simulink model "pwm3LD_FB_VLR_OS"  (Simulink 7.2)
settings: Solver=ode3  SolverMode=SingleTasking  StartTime=0.0  StopTime=0.1  FixedStep=10e-6  MaxStep=1e-4  RelTol=1e-3
PreLoadFcn:
  | INIT_PWM_3L

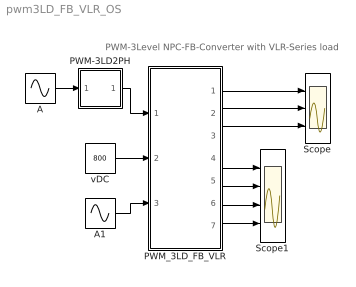
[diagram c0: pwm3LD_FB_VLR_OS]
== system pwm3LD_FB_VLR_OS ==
  note: PWM-3Level NPC-FB-Converter with VLR-Series load
  A : Sin  Amplitude=.8  Frequency=2*pi*50  Phase=[0 ]  SampleTime=0
  A1 : Sin  Amplitude=200  Frequency=2*pi*50  Phase=[0 ]  SampleTime=0
  PWM-3LD2PH : Subsystem  mask(PWM-3LD_3PH){FT=900, PHT=0, A=0.5, O1=0.5, O2=-0.5, DT=1e-6}
      mask prompts: FT "Frequency of Trian Sig."; PHT "Phase Angle of Trian. Sig."; A "Amplitude of Trian. Sig."; O1 "Offset of 1st Trian"; O2 "Offset of 2nd Trian."; DT "Dead Time"
      mask help: Pulse Width Modulation for 2 Legs of 3 Level Neutral point clamped Converter
  PWM_3LD_FB_VLR : Subsystem  mask(pwm_3LD_FB_VLR_OS){RL=1, LL=1e-3}
      mask prompts: RL "Load Resistance"; LL "Load Inductance"
      mask help: Open Source 3-Level NPC Full Bridge Converter with VLR load Input Vector u: u[0]= L3L1_TD1.gate u[1]= L3L1_TD2.gate u[2]= L3L1_TD3.gate u[3]= L3L1_TD4.gate u[4]= L3L2_TD1.gate u[5]= L3L2_TD2.gate u[6]= L3L2_TD3.gate u[7]= L3L2_TD4.gate u[8]= VDC u[9]= EL Output Vector y: y[0]= Va.v, Output AC Voltage to middle point y[1]= Ia.I, Output AC Current y[2]= Vab.V, Output AC Voltage y[3]= T1.I y[4]= D1.I y[5]= T1.V y[6]= T2.I y[7]= D2.I y[8]= T2.V y[9]= D5.I y[10]= D5.V y[11]= IDC1, Input DC Current y[12]= IDC2, Input DC Current Parameter Vector p: p[0]=RL p[1]=LL You can pause the simulation during 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
  Scope : Scope  NumInputPorts=3
  Scope1 : Scope  NumInputPorts=4
  vDC : Constant  Value=800  OutDataType=sfix(16)  OutScaling=2^0
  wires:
  A/1 -> PWM-3LD2PH/1(In1)
  vDC/1 -> PWM_3LD_FB_VLR/2(vDC)
  A1/1 -> PWM_3LD_FB_VLR/3(E_A)
  PWM-3LD2PH/1(Out1) -> PWM_3LD_FB_VLR/1(Sw)
  PWM_3LD_FB_VLR/4("iT1, iD1,vT1") -> Scope1/1
  PWM_3LD_FB_VLR/5("iT2, iD2,vT2") -> Scope1/2
  PWM_3LD_FB_VLR/6(iD5,vD5) -> Scope1/3
  PWM_3LD_FB_VLR/7(iDC1,iDC2) -> Scope1/4
  PWM_3LD_FB_VLR/1(vA) -> Scope/1
  PWM_3LD_FB_VLR/2(iA) -> Scope/2
  PWM_3LD_FB_VLR/3(vAB) -> Scope/3

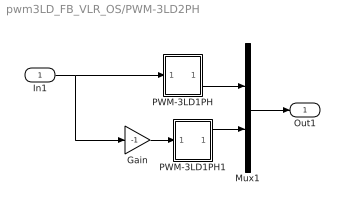
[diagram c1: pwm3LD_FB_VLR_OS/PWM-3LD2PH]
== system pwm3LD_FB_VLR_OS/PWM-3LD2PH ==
  In1 : Inport  OutDataType=sfix(16)  OutScaling=2^0
  Gain : Gain  Gain=-1  ParameterDataType=sfix(16)  ParameterScaling=2^0  OutDataType=sfix(16)  OutScaling=2^0
  Mux1 : Mux  Inputs=2
  PWM-3LD1PH : Subsystem  mask(PWM-3LD1PH){FT=FT, PHT=PHT, A=A, O1=O1, O2=O2, DT=DT}
      mask prompts: FT "Frequency of Trian Sig."; PHT "Phase Angle of Trian. Sig."; A "Amplitude of Trian. Sig."; O1 "Offset of 1st Trian"; O2 "Offset of 2nd Trian."; DT "Dead Time"
      mask help: Pulse Width Modulation for 1 Phase 3 Level Floating Capacitor Converter
  PWM-3LD1PH1 : Subsystem  mask(PWM-3LD1PH){FT=FT, PHT=PHT, A=A, O1=O1, O2=O2, DT=DT}
      mask prompts: FT "Frequency of Trian Sig."; PHT "Phase Angle of Trian. Sig."; A "Amplitude of Trian. Sig."; O1 "Offset of 1st Trian"; O2 "Offset of 2nd Trian."; DT "Dead Time"
      mask help: Pulse Width Modulation for 1 Phase 3 Level Floating Capacitor Converter
  Out1 : Outport
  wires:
  PWM-3LD1PH1/1(Out1) -> Mux1/2
  PWM-3LD1PH/1(Out1) -> Mux1/1
  In1/1 -> Gain/1, PWM-3LD1PH/1(In1)
  Gain/1 -> PWM-3LD1PH1/1(In1)
  Mux1/1 -> Out1/1

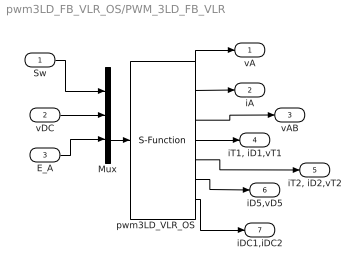
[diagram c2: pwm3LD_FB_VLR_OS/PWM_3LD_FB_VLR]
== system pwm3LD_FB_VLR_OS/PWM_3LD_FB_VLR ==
  Sw : Inport  OutDataType=sfix(16)  OutScaling=2^0
  vDC : Inport  Port=2  OutDataType=sfix(16)  OutScaling=2^0
  E_A : Inport  Port=3  OutDataType=sfix(16)  OutScaling=2^0
  Mux : Mux  Inputs="[8  1  1]"
  pwm3LD_VLR_OS : S-Function  FunctionName=s_pwm_3LD_FB_VLR_OS  Parameters="[RL  LL]"  EnableBusSupport=off
  vA : Outport  OutDataType=sfix(16)  OutScaling=2^0
  iA : Outport  Port=2  OutDataType=sfix(16)  OutScaling=2^0
  vAB : Outport  Port=3  OutDataType=sfix(16)  OutScaling=2^0
  "iT1, iD1,vT1" : Outport  Port=4  OutDataType=sfix(16)  OutScaling=2^0
  "iT2, iD2,vT2" : Outport  Port=5  OutDataType=sfix(16)  OutScaling=2^0
  iD5,vD5 : Outport  Port=6  OutDataType=sfix(16)  OutScaling=2^0
  iDC1,iDC2 : Outport  Port=7  OutDataType=sfix(16)  OutScaling=2^0
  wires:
  Sw/1 -> Mux/1
  vDC/1 -> Mux/2
  Mux/1 -> pwm3LD_VLR_OS/1
  E_A/1 -> Mux/3
  pwm3LD_VLR_OS/1 -> vA/1
  pwm3LD_VLR_OS/2 -> iA/1
  pwm3LD_VLR_OS/3 -> vAB/1
  pwm3LD_VLR_OS/4 -> "iT1, iD1,vT1"/1
  pwm3LD_VLR_OS/5 -> "iT2, iD2,vT2"/1
  pwm3LD_VLR_OS/6 -> iD5,vD5/1
  pwm3LD_VLR_OS/7 -> iDC1,iDC2/1

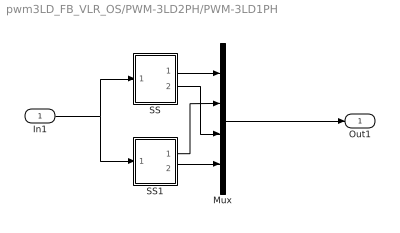
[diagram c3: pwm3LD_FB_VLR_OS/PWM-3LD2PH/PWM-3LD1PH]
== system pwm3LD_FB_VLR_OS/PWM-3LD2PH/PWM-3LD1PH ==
  In1 : Inport  OutDataType=sfix(16)  OutScaling=2^0
  Mux : Mux
  SS : Subsystem
  SS1 : Subsystem
  Out1 : Outport
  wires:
  In1/1 -> SS1/1(I1), SS/1(I1)
  SS1/1(O1) -> Mux/2
  SS/2(O2) -> Mux/3
  Mux/1 -> Out1/1
  SS/1(O1) -> Mux/1
  SS1/2(O2) -> Mux/4

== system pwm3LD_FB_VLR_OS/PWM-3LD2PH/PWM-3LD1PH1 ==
  In1 : Inport  OutDataType=sfix(16)  OutScaling=2^0
  Mux : Mux
  SS : Subsystem
  SS1 : Subsystem
  Out1 : Outport
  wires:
  SS1/2(O2) -> Mux/4
  SS/1(O1) -> Mux/1
  Mux/1 -> Out1/1
  SS/2(O2) -> Mux/3
  SS1/1(O1) -> Mux/2
  In1/1 -> SS/1(I1), SS1/1(I1)

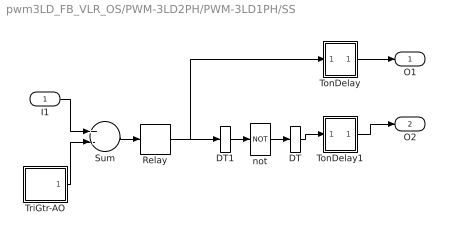
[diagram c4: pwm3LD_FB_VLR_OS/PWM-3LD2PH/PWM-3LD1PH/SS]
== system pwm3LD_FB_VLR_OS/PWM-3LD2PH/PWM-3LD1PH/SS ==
  I1 : Inport  OutDataType=sfix(16)  OutScaling=2^0
  DT : DataTypeConversion
  DT1 : DataTypeConversion
  Relay : Relay  OutDataType=sfix(16)  OutScaling=2^0
  Sum : Sum  Inputs=+-  OutDataType=sfix(16)  OutScaling=2^0
  TonDelay : Subsystem  mask(TonDelay){DT=DT}
      mask prompts: DT "Dead Time"
      mask help: Turn on dead time to protect against short circuit of the converter leg
  TonDelay1 : Subsystem  mask(TonDelay){DT=DT}
      mask prompts: DT "Dead Time"
      mask help: Turn on dead time to protect against short circuit of the converter leg
  TriGtr-AO : Subsystem  mask(TriGtr-AO){A=A, O=O1, T=1/FT, Td=PHT/FT/180}
      mask prompts: A "Amplitude"; O "Offset"; T "Period Time"; Td "Time Delay"
      mask help: Triangular Wave Generator with variable time delay, variable amplitude and offset
  not : Logic  Operator=NOT  Inputs=1
  O1 : Outport  InitialOutput=0
  O2 : Outport  Port=2  InitialOutput=0
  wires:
  TonDelay/1(s1d) -> O1/1
  Relay/1 -> TonDelay/1(s1), DT1/1
  TonDelay1/1(s1d) -> O2/1
  not/1 -> DT/1
  Sum/1 -> Relay/1
  TriGtr-AO/1(Out1) -> Sum/2
  I1/1 -> Sum/1
  DT/1 -> TonDelay1/1(s1)
  DT1/1 -> not/1

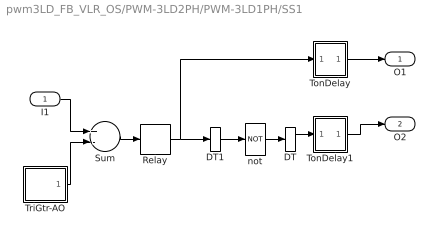
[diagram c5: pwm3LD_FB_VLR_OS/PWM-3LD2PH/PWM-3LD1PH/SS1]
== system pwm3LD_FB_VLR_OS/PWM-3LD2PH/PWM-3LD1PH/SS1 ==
  I1 : Inport  OutDataType=sfix(16)  OutScaling=2^0
  DT : DataTypeConversion
  DT1 : DataTypeConversion
  Relay : Relay  OutDataType=sfix(16)  OutScaling=2^0
  Sum : Sum  Inputs=+-  OutDataType=sfix(16)  OutScaling=2^0
  TonDelay : Subsystem  mask(TonDelay){DT=DT}
      mask prompts: DT "Dead Time"
      mask help: Turn on dead time to protect against short circuit of the converter leg
  TonDelay1 : Subsystem  mask(TonDelay){DT=DT}
      mask prompts: DT "Dead Time"
      mask help: Turn on dead time to protect against short circuit of the converter leg
  TriGtr-AO : Subsystem  mask(TriGtr-AO){A=A, O=O2, T=1/FT, Td=PHT/FT/180}
      mask prompts: A "Amplitude"; O "Offset"; T "Period Time"; Td "Time Delay"
      mask help: Triangular Wave Generator with variable time delay, variable amplitude and offset
  not : Logic  Operator=NOT  Inputs=1
  O1 : Outport  InitialOutput=0
  O2 : Outport  Port=2  InitialOutput=0
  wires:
  TonDelay/1(s1d) -> O1/1
  Relay/1 -> TonDelay/1(s1), DT1/1
  TonDelay1/1(s1d) -> O2/1
  not/1 -> DT/1
  Sum/1 -> Relay/1
  TriGtr-AO/1(Out1) -> Sum/2
  I1/1 -> Sum/1
  DT/1 -> TonDelay1/1(s1)
  DT1/1 -> not/1

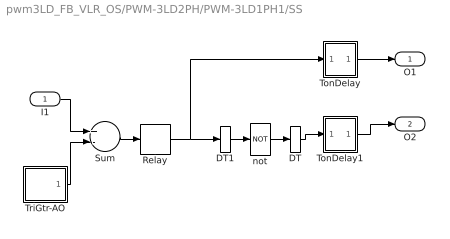
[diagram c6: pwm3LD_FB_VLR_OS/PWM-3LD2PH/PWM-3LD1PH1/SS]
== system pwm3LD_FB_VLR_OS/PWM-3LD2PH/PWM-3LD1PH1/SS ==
  I1 : Inport  OutDataType=sfix(16)  OutScaling=2^0
  DT : DataTypeConversion
  DT1 : DataTypeConversion
  Relay : Relay  OutDataType=sfix(16)  OutScaling=2^0
  Sum : Sum  Inputs=+-  OutDataType=sfix(16)  OutScaling=2^0
  TonDelay : Subsystem  mask(TonDelay){DT=DT}
      mask prompts: DT "Dead Time"
      mask help: Turn on dead time to protect against short circuit of the converter leg
  TonDelay1 : Subsystem  mask(TonDelay){DT=DT}
      mask prompts: DT "Dead Time"
      mask help: Turn on dead time to protect against short circuit of the converter leg
  TriGtr-AO : Subsystem  mask(TriGtr-AO){A=A, O=O1, T=1/FT, Td=PHT/FT/180}
      mask prompts: A "Amplitude"; O "Offset"; T "Period Time"; Td "Time Delay"
      mask help: Triangular Wave Generator with variable time delay, variable amplitude and offset
  not : Logic  Operator=NOT  Inputs=1
  O1 : Outport  InitialOutput=0
  O2 : Outport  Port=2  InitialOutput=0
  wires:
  DT1/1 -> not/1
  DT/1 -> TonDelay1/1(s1)
  I1/1 -> Sum/1
  TriGtr-AO/1(Out1) -> Sum/2
  Sum/1 -> Relay/1
  not/1 -> DT/1
  TonDelay1/1(s1d) -> O2/1
  Relay/1 -> DT1/1, TonDelay/1(s1)
  TonDelay/1(s1d) -> O1/1

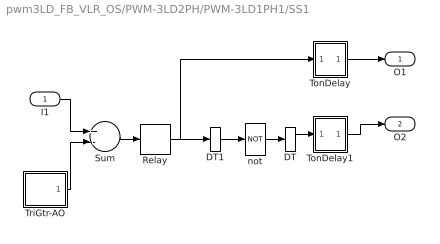
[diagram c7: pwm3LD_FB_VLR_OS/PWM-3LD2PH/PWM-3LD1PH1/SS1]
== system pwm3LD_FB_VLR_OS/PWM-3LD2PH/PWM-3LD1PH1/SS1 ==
  I1 : Inport  OutDataType=sfix(16)  OutScaling=2^0
  DT : DataTypeConversion
  DT1 : DataTypeConversion
  Relay : Relay  OutDataType=sfix(16)  OutScaling=2^0
  Sum : Sum  Inputs=+-  OutDataType=sfix(16)  OutScaling=2^0
  TonDelay : Subsystem  mask(TonDelay){DT=DT}
      mask prompts: DT "Dead Time"
      mask help: Turn on dead time to protect against short circuit of the converter leg
  TonDelay1 : Subsystem  mask(TonDelay){DT=DT}
      mask prompts: DT "Dead Time"
      mask help: Turn on dead time to protect against short circuit of the converter leg
  TriGtr-AO : Subsystem  mask(TriGtr-AO){A=A, O=O2, T=1/FT, Td=PHT/FT/180}
      mask prompts: A "Amplitude"; O "Offset"; T "Period Time"; Td "Time Delay"
      mask help: Triangular Wave Generator with variable time delay, variable amplitude and offset
  not : Logic  Operator=NOT  Inputs=1
  O1 : Outport  InitialOutput=0
  O2 : Outport  Port=2  InitialOutput=0
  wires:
  DT1/1 -> not/1
  DT/1 -> TonDelay1/1(s1)
  I1/1 -> Sum/1
  TriGtr-AO/1(Out1) -> Sum/2
  Sum/1 -> Relay/1
  not/1 -> DT/1
  TonDelay1/1(s1d) -> O2/1
  Relay/1 -> DT1/1, TonDelay/1(s1)
  TonDelay/1(s1d) -> O1/1

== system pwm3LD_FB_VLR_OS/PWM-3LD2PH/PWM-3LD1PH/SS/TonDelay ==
  s1 : Inport  Orientation=down  OutDataType=sfix(16)  OutScaling=2^0
  Int : Integrator  ExternalReset=falling
  Rel1 : Relay  OnSwitchValue=DT  OutDataType=sfix(16)  OutScaling=2^0
  s1d : Outport  InitialOutput=0
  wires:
  Rel1/1 -> s1d/1
  s1/1 -> Int/1, Int/2
  Int/1 -> Rel1/1

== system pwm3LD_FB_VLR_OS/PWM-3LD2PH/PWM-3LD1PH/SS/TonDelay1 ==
  s1 : Inport  Orientation=down  OutDataType=sfix(16)  OutScaling=2^0
  Int : Integrator  ExternalReset=falling
  Rel1 : Relay  OnSwitchValue=DT  OutDataType=sfix(16)  OutScaling=2^0
  s1d : Outport  InitialOutput=0
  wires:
  Rel1/1 -> s1d/1
  s1/1 -> Int/1, Int/2
  Int/1 -> Rel1/1

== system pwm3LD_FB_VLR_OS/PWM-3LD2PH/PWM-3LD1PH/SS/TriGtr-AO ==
  Ampl. : Gain  Gain=A  ParameterDataType=sfix(16)  ParameterScaling=2^0  OutDataType=sfix(16)  OutScaling=2^0
  Offset : Constant  Value=O  OutDataType=sfix(16)  OutScaling=2^0
  Sum : Sum  OutDataType=sfix(16)  OutScaling=2^0
  TriGtr : Subsystem  mask(TriGtr){T=1/FT, Td=PHT/FT/180}
      mask prompts: T "Period Time"; Td "Time Delay"
      mask help: Triangular Wave Generator with variable time delay
  Out1 : Outport
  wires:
  Sum/1 -> Out1/1
  Ampl./1 -> Sum/1
  TriGtr/1(O) -> Ampl./1
  Offset/1 -> Sum/2

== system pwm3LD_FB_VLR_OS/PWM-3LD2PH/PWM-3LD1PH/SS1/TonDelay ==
  s1 : Inport  Orientation=down  OutDataType=sfix(16)  OutScaling=2^0
  Int : Integrator  ExternalReset=falling
  Rel1 : Relay  OnSwitchValue=DT  OutDataType=sfix(16)  OutScaling=2^0
  s1d : Outport  InitialOutput=0
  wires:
  Rel1/1 -> s1d/1
  s1/1 -> Int/1, Int/2
  Int/1 -> Rel1/1

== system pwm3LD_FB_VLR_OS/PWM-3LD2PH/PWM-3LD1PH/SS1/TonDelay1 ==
  s1 : Inport  Orientation=down  OutDataType=sfix(16)  OutScaling=2^0
  Int : Integrator  ExternalReset=falling
  Rel1 : Relay  OnSwitchValue=DT  OutDataType=sfix(16)  OutScaling=2^0
  s1d : Outport  InitialOutput=0
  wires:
  Rel1/1 -> s1d/1
  s1/1 -> Int/1, Int/2
  Int/1 -> Rel1/1

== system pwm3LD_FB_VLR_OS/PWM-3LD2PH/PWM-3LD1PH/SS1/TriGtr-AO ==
  Ampl. : Gain  Gain=A  ParameterDataType=sfix(16)  ParameterScaling=2^0  OutDataType=sfix(16)  OutScaling=2^0
  Offset : Constant  Value=O  OutDataType=sfix(16)  OutScaling=2^0
  Sum : Sum  OutDataType=sfix(16)  OutScaling=2^0
  TriGtr1 : Subsystem  mask(TriGtr){T=1/FT, Td=PHT/FT/180}
      mask prompts: T "Period Time"; Td "Time Delay"
      mask help: Triangular Wave Generator with variable time delay
  Out1 : Outport
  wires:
  Offset/1 -> Sum/2
  TriGtr1/1(O) -> Ampl./1
  Ampl./1 -> Sum/1
  Sum/1 -> Out1/1

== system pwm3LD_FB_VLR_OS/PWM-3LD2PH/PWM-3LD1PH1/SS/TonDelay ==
  s1 : Inport  Orientation=down  OutDataType=sfix(16)  OutScaling=2^0
  Int : Integrator  ExternalReset=falling
  Rel1 : Relay  OnSwitchValue=DT  OutDataType=sfix(16)  OutScaling=2^0
  s1d : Outport  InitialOutput=0
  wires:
  Int/1 -> Rel1/1
  s1/1 -> Int/2, Int/1
  Rel1/1 -> s1d/1

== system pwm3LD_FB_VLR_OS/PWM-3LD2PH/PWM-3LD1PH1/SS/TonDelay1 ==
  s1 : Inport  Orientation=down  OutDataType=sfix(16)  OutScaling=2^0
  Int : Integrator  ExternalReset=falling
  Rel1 : Relay  OnSwitchValue=DT  OutDataType=sfix(16)  OutScaling=2^0
  s1d : Outport  InitialOutput=0
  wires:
  Int/1 -> Rel1/1
  s1/1 -> Int/2, Int/1
  Rel1/1 -> s1d/1

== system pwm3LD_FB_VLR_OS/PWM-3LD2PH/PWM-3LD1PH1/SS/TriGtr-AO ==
  Ampl. : Gain  Gain=A  ParameterDataType=sfix(16)  ParameterScaling=2^0  OutDataType=sfix(16)  OutScaling=2^0
  Offset : Constant  Value=O  OutDataType=sfix(16)  OutScaling=2^0
  Sum : Sum  OutDataType=sfix(16)  OutScaling=2^0
  TriGtr : Subsystem  mask(TriGtr){T=1/FT, Td=PHT/FT/180}
      mask prompts: T "Period Time"; Td "Time Delay"
      mask help: Triangular Wave Generator with variable time delay
  Out1 : Outport
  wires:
  Offset/1 -> Sum/2
  TriGtr/1(O) -> Ampl./1
  Ampl./1 -> Sum/1
  Sum/1 -> Out1/1

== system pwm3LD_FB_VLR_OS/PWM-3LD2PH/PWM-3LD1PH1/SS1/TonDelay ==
  s1 : Inport  Orientation=down  OutDataType=sfix(16)  OutScaling=2^0
  Int : Integrator  ExternalReset=falling
  Rel1 : Relay  OnSwitchValue=DT  OutDataType=sfix(16)  OutScaling=2^0
  s1d : Outport  InitialOutput=0
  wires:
  Int/1 -> Rel1/1
  s1/1 -> Int/2, Int/1
  Rel1/1 -> s1d/1

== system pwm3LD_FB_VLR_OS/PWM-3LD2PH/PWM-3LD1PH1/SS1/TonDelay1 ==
  s1 : Inport  Orientation=down  OutDataType=sfix(16)  OutScaling=2^0
  Int : Integrator  ExternalReset=falling
  Rel1 : Relay  OnSwitchValue=DT  OutDataType=sfix(16)  OutScaling=2^0
  s1d : Outport  InitialOutput=0
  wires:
  Int/1 -> Rel1/1
  s1/1 -> Int/2, Int/1
  Rel1/1 -> s1d/1

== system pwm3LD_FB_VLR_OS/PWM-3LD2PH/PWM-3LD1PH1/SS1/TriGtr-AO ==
  Ampl. : Gain  Gain=A  ParameterDataType=sfix(16)  ParameterScaling=2^0  OutDataType=sfix(16)  OutScaling=2^0
  Offset : Constant  Value=O  OutDataType=sfix(16)  OutScaling=2^0
  Sum : Sum  OutDataType=sfix(16)  OutScaling=2^0
  TriGtr : Subsystem  mask(TriGtr){T=1/FT, Td=PHT/FT/180}
      mask prompts: T "Period Time"; Td "Time Delay"
      mask help: Triangular Wave Generator with variable time delay
  Out1 : Outport
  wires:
  Sum/1 -> Out1/1
  Ampl./1 -> Sum/1
  TriGtr/1(O) -> Ampl./1
  Offset/1 -> Sum/2

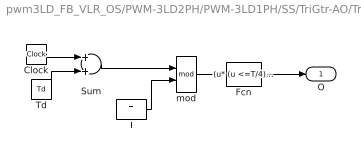
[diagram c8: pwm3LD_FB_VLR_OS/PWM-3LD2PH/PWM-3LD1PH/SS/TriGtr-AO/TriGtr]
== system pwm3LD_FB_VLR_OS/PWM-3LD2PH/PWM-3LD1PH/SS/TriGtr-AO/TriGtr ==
  Clock : Clock
  Fcn : Fcn  Expr="(u* (u <=T/4) * 4/T)   +  (  (u > T/4) && ( u <=3*T/4) )* ( 1 - (u-T/4) *4/T )   +  ( (u > 3*T/4)&& (u<=T)) * ( ((u -3*T/4)* 4/T )-1 )"
  Sum : Sum
  T : Constant  Value=T
  Td : Constant  Value=Td
  mod : Math  Operator=mod
  O : Outport  InitialOutput=0
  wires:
  mod/1 -> Fcn/1
  Fcn/1 -> O/1
  Clock/1 -> Sum/1
  T/1 -> mod/2
  Sum/1 -> mod/1
  Td/1 -> Sum/2

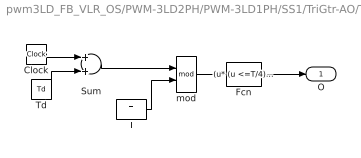
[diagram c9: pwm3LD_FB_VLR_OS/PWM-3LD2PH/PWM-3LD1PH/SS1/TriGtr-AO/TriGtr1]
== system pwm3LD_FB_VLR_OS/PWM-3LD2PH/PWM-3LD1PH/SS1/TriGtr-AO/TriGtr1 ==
  Clock : Clock
  Fcn : Fcn  Expr="(u* (u <=T/4) * 4/T)   +  (  (u > T/4) && ( u <=3*T/4) )* ( 1 - (u-T/4) *4/T )   +  ( (u > 3*T/4)&& (u<=T)) * ( ((u -3*T/4)* 4/T )-1 )"
  Sum : Sum
  T : Constant  Value=T
  Td : Constant  Value=Td
  mod : Math  Operator=mod
  O : Outport  InitialOutput=0
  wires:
  Td/1 -> Sum/2
  Sum/1 -> mod/1
  T/1 -> mod/2
  Clock/1 -> Sum/1
  Fcn/1 -> O/1
  mod/1 -> Fcn/1

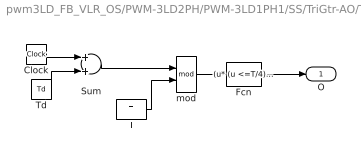
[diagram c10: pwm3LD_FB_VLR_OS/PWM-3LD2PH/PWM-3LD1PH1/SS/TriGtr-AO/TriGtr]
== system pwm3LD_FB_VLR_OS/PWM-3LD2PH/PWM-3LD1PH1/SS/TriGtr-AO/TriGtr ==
  Clock : Clock
  Fcn : Fcn  Expr="(u* (u <=T/4) * 4/T)   +  (  (u > T/4) && ( u <=3*T/4) )* ( 1 - (u-T/4) *4/T )   +  ( (u > 3*T/4)&& (u<=T)) * ( ((u -3*T/4)* 4/T )-1 )"
  Sum : Sum
  T : Constant  Value=T
  Td : Constant  Value=Td
  mod : Math  Operator=mod
  O : Outport  InitialOutput=0
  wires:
  Td/1 -> Sum/2
  Sum/1 -> mod/1
  T/1 -> mod/2
  Clock/1 -> Sum/1
  Fcn/1 -> O/1
  mod/1 -> Fcn/1

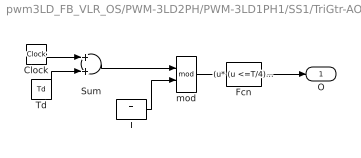
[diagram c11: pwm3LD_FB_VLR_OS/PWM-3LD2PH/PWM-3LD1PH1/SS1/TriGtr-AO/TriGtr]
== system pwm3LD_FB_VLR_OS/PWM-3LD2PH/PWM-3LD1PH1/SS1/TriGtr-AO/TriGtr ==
  Clock : Clock
  Fcn : Fcn  Expr="(u* (u <=T/4) * 4/T)   +  (  (u > T/4) && ( u <=3*T/4) )* ( 1 - (u-T/4) *4/T )   +  ( (u > 3*T/4)&& (u<=T)) * ( ((u -3*T/4)* 4/T )-1 )"
  Sum : Sum
  T : Constant  Value=T
  Td : Constant  Value=Td
  mod : Math  Operator=mod
  O : Outport  InitialOutput=0
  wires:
  Td/1 -> Sum/2
  Sum/1 -> mod/1
  T/1 -> mod/2
  Clock/1 -> Sum/1
  Fcn/1 -> O/1
  mod/1 -> Fcn/1
